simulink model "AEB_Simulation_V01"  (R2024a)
settings: Solver=ode23tb  StartTime=0.0  StopTime=inf  RelTol=2e-1
PreLoadFcn:
  | helperCreateDetectorBus;
model workspace (MAT data in the model file):
  EngPwr = 352122.842504
  EngWc = 4.047
  Tdiff = 849
  Tlim = 1000
  VEH : object (value not decoded)
undefined symbols (not defined in the file or in its folder): automotive_project_windows, blkdiag, C, car, D, Female, MATLAB, Performance, R2024a, Row, shared, sim3d_projects, Sim3dSensor, toolbox, UE, vector, VehicleSimulation, WindowsNoEditor
libraries: simulink x7, sim3dautolib x4, vehdynlibtirecommon x4, autolibutils x4, sharedtransform x2, sim3dcameralib x1, sim3dphyssensorlib x1, sim3dlib x1, motalgorithmslib x1, vehdynlibtire x1, vehdynlibsteering x1, autolibshared x1
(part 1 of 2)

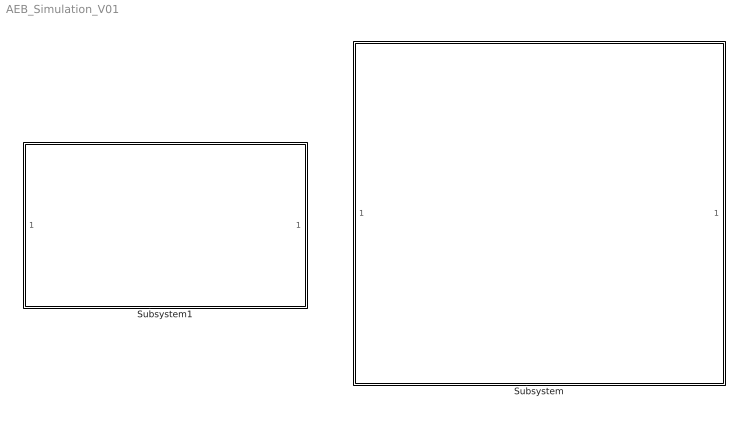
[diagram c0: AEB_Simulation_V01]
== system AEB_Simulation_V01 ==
  Subsystem : Subsystem
  Subsystem1 : Subsystem

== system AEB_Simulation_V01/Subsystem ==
  note: LED-Strip
  note: Controls
  {1..5} (5 alike) : LampBlock  LabelPosition=Hide
  Deceleration / Acceleration : SliderBlock  LabelPosition=Hide  ScaleMin=-1  ScaleMax=1  TickInterval=.25
  Direction : RotarySwitchBlock  LabelPosition=Hide
  Steering : KnobBlock  LabelPosition=Hide  ScaleMin=-400  ScaleMax=400  TickInterval=100
  Velocity : LinearGaugeBlock  LabelPosition=Hide  ScaleMax=30  TickInterval=5

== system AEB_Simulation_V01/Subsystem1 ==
  3D-Simulation : Subsystem
  AEB : Display
  BB-Detection and Tracking : Subsystem  Commented=on
  EGO : Subsystem
  MIO Detection : Subsystem  Commented=on
  Manual Switch : ManualSwitch  CurrentSetting=0
  Subsystem : Subsystem
  Terminator : Terminator
  Terminator1 : Terminator
  Terminator2 : Terminator
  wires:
  EGO/1(EGO_Position) -> 3D-Simulation/1(In1)
  Manual Switch/1 -> EGO/1(AEB), AEB/1
  MIO Detection/2(Relative Velocity) -> Terminator/1
  MIO Detection/4(MIO Track) -> Terminator2/1
  MIO Detection/3(Relative Distance) -> Terminator1/1
  MIO Detection/1(AEB) -> Manual Switch/1
  BB-Detection and Tracking/1(confirmedTracks) -> MIO Detection/1(confirmedTracks)
  3D-Simulation/1(lidar) -> Subsystem/1(In1), BB-Detection and Tracking/1(lidar)
  Subsystem/1(Out1) -> Manual Switch/2

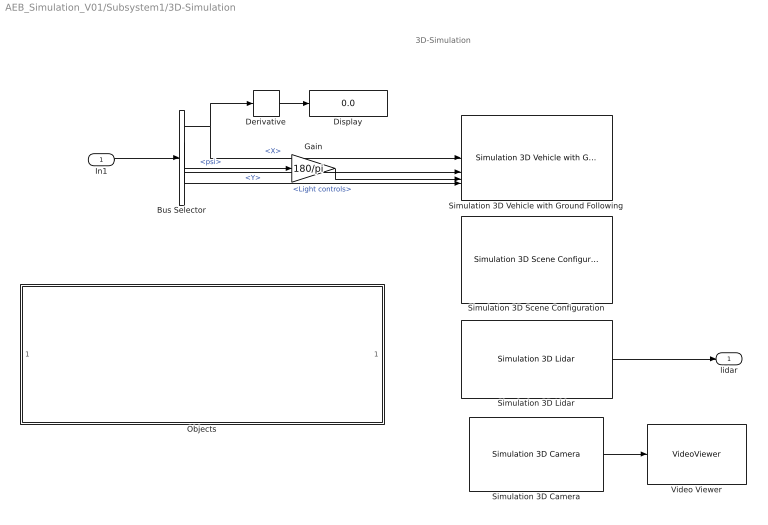
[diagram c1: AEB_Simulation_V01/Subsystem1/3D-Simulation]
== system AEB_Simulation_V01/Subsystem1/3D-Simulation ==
  note: 3D-Simulation
  In1 : Inport
  Bus Selector : BusSelector  OutputSignals=VehFdbk.InertFrm.Cg.Disp.X,VehFdbk.InertFrm.Cg.Disp.Y,VehFdbk.InertFrm.Cg.Ang.psi,Light controls
  Derivative : Derivative
  Display : Display
  Gain : Gain  Gain=180/pi
  Objects : Subsystem
  Simulation 3D Camera : sim3dcameralib/Simulation 3D Camera  Priority=1  sensorTag=Sim3dSensor�  sensorId=3  sensorName=Sim3dSensor�  vehTagList={'Scene Origin';'SimulinkVehicle1';'SimulinkVehicle2'}  vehTag=SimulinkVehicle1  mountLoc=Hood center  offsetFlag=on  tmountOffset=[-1.1, 0, 0.3]  extTmount=off  rmountOffset=[0, 5, 0]  extRmount=off  FocalLength=[1109, 1109]  OpticalCenter=[640, 360]  ImageSize=[720, 1280]  RadialDistortion=[0, 0]  TangentialDistortion=[0, 0]  SensorSkew=0  DepthOutportEnabled=off  SemanticOutportEnabled=off  TransformOutportEnabled=off  SampleTime=-1  mountPoint=[0.363999992609024 0 1.39999997615814]  mountOrientation=[0 -5 0]  aMode=3  ID=3
  Simulation 3D Lidar : sim3dphyssensorlib/Simulation 3D Lidar  Priority=1  sensorTag=Sim3dSensor�  sensorId=1  sensorName=Sim3dSensor�  vehTagList={'Scene Origin';'SimulinkVehicle1'}  vehTag=SimulinkVehicle1  mountLoc=Roof center  offsetFlag=off  tmountOffset=[0, 0, 0]  rmountOffset=[0, 0, 0]  DetectionRange=120  RangeResolution=0.02  VerticalFOV=40  VerticalResolution=1.25  HorizontalFOV=60  HorizontalResolution=0.16  DistanceOutportEnabled=off  ReflectivityOutportEnabled=off  SemanticOutportEnabled=off  TransformOutportEnabled=off  SampleTime=-1  mountPoint=[-0.449999988079071 0 1.67999994754791]  mountOrientation=[0 0 0]  aMode=3  ID=1
  Simulation 3D Scene Configuration : sim3dlib/Simulation 3D Scene Configuration  Priority=0  ProjectFormat=Default Scenes  SceneDesc=Parking lot  ProjectName=C:\MATLAB\R2024a\toolbox\shared\sim3d_projects\automotive_project_windows\UE\WindowsNoEditor\VehicleSimulation.exe  ScenePath=/Game/Maps/HwStrght  EnableOpenDRIVE=off  vehTagList={'Custom';'Scene Origin';'SimulinkVehicle1';'SimulinkVehicle2'}  vehTag=SimulinkVehicle1  FreeCameraInitialTranslation=[0, 0, 0]  FreeCameraDefaultInitialTranslation=[-6, 0, 2]  FreeCameraInitialRotation=[0, 0, 0]  FreeCameraDefaultInitialRotation=[0, -15, 0]  OpVisEn=off  Ts=0.1  EnableWindow=off  EnableRemoteAccess=off  EnableWeather=off  SunAzimuth=90  SunAltitude=40.0  EnableGeospatialSun=off  Latitude=0  Longitude=0  Date=2023-01-01  Time=10:30:00  GeoTimeZone=-5.0  SunDaylightSaving=off  wind=1  clouds=10  EnableVolumetricClouds=off  CloudCoverage=0  CloudAltitude=6  fog=0  rain=0  RaindropsEffect=off  SnowDensity=0  EnableGeospatial=off  UseTrueOrigin=off  OriginHeight=200  OriginLatitude=40.744652  OriginLongitude=-73.988864  MapStyle=Aerial  AdditionalAssetIDs=[]  UseAdvancedSunSky=off  SolarTime=11  TimeZone=-5  Day=21  Month=9  Year=2022  UseDaylightSavingTime=on  DSTStartDay=10  DSTStartMonth=3  DSTEndDay=3  DSTEndMonth=11  DSTSwitchHour=2  sensorTag=MainCamera1  sensorId=1  sensorName=MainCamera1  mountLoc=Origin  offsetFlag=off  tmountOffset=[0, 0, 0]  rmountOffset=[0, 0, 0]  HorizontalResolution=1280  VerticalResolution=720  HorizontalFOV=60  mountPoint=[0 0 0]  mountOrientation=[0 0 0]  aMode=3  ID=1  GeoTrigger=Inactive
  Simulation 3D Vehicle with Ground Following : sim3dautolib/Simulation 3D Vehicle with Ground Following  Priority=-1  PassVehMesh=Sedan  MeshPath=/MathWorksAutomotiveContent/Vehicles/Muscle/Meshes/SK_MuscleCar.SK_MuscleCar  TrackWidth=1.9  WheelBase=3  WheelRadius=0.35  VehColor=Red  InitialPos=[0, 0, 0]  InitialRot=[0, 0, 0]  ActorName=SimulinkVehicle1  SampleTime=-1  ActorType=SimulinkVehicle  ID=1  aMode=3  ActorTag=SimulinkVehicle1  CoordinateScheme=ISO  VehLightsControl=on  HeadlightColor=[ 1, 1, 1 ]  HighBeamIntensity=100000  LowBeamIntensity=60000  HighBeamConeAngle=70  LowBeamConeAngle=70  LeftHeadlightOrientation=[ 0, 0 ]  RightHeadlightOrientation=[ 0, 0 ]  BrakelightIntensity=500  ReverselightIntensity=500  SignallightIntensity=500  SignallightPeriod=1  SignalPulseWidth=50  TransformOutportEnabled=off
  Video Viewer : VideoViewer  FigPos=[593 850 943.333333333333 495.333333333333]
  lidar : Outport
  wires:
  Bus Selector/3 -> Gain/1  "<psi>"
  Bus Selector/2 -> Simulation 3D Vehicle with Ground Following/2  "<Y>"
  Bus Selector/4 -> Simulation 3D Vehicle with Ground Following/4  "<Light controls>"
  Simulation 3D Lidar/1 -> lidar/1
  Bus Selector/1 -> Derivative/1, Simulation 3D Vehicle with Ground Following/1  "<X>"
  In1/1 -> Bus Selector/1
  Gain/1 -> Simulation 3D Vehicle with Ground Following/3
  Derivative/1 -> Display/1
  Simulation 3D Camera/1 -> Video Viewer/1

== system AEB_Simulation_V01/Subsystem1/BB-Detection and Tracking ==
  note: Copyright 2019-2020 The MathWorks, Inc.
  note: Visualization
  note: Tracking Algorithm
  note: Lidar Segmentation and Clustering
  lidar : Inport
  Bounding Box Detector : MATLABSystem  System=HelperBoundingBoxDetectorBlock  DetectionBusName=detectionBus  SegmentationBusName=segmentationBus  NumLidarPoints=55000  XLimits=[ -70, 70 ]  YLimits=[ -6, 6 ]  ZLimits=[ -2, 10 ]  GroundMaxDistance=0.3  GroundReferenceVector=[ 0, 0, 1 ]  GroundMaxAngularDistance=5  SegmentationMinDistance=1.8  MinDetectionsPerCluster=1  MaxZDistanceCluster=3  MinZDistanceCluster=-3  EgoVehicleRadius=3  MeasurementNoise=blkdiag( 0.25*eye( 3 ), 25, eye( 3 ) )  MeasurementParameters="{  }"  SimulateUsing=Interpreted execution
  Calculate Detectability : MATLAB Function  TreatAsAtomicUnit=on
  Constant : Constant  Value=[1 3 6]
  Delay : Delay  DelayLength=1
  Terminator : Terminator
  Tracker : motalgorithmslib/Joint Probabilistic Data Association Multi Object Tracker  TrackerIndex=uint32( 0 )  FilterInitializationFcn=helperInitIMMFilter  MaxNumEvents=inf  EventGenerationFcn=jpdaEvents  MaxNumTracks=100  MaxNumSensors=20  TimeTolerance=1e-5  OOSMHandling=Terminate  MaxNumOOSMSteps=3  StateParametersSimulink=struct  HasStateParametersInput=off  EnableMemoryManagement=off  SimulateUsing=Interpreted execution  AssignmentThreshold=[75 1000]  InitializationThreshold=0  DetectionProbability=0.9  ClutterDensity=1e-9  TrackLogic=History  pHistoryConfThreshold=[7 10]  pHistoryDelThreshold=[8 10]  pIntegratedConfThreshold=0.95  pIntegratedDelThreshold=0.1  HitMissThreshold=0.1  NewTargetDensity=1e-5  DeathRate=0.01  TimeInputSource=Input port  HasCostMatrixInput=off  HasDetectableTrackIDsInput=on  TentativeTracksOutputPort=off  AllTracksOutputPort=on  InfoOutputPort=off  BusNameSource=Property  BusName=trackBus  BusName2Source=Auto  BusName2=BusTrackerInfo  MaxNumDetectionsPerSensor=100  MaxNumDetectionsPerCluster=5  MaxNumTracksPerCluster=5  ClusterViolationHandling=Split and warn
  Visualization : MATLABSystem  Commented=on  System=HelperLidarExampleDisplayBlock  LidarDataReaderBlockName=Lidar Data Reader  ImageDataReaderBlockName=Image Data Reader  DetectorBlockName=Bounding Box Detector  TrackerBlockName=Tracker  PositionIndex=[ 1, 3, 6 ]  VelocityIndex=[ 2, 4, 7 ]  DimensionIndex=[9 10 11]  YawIndex=8  RecordGIF=true  MovieName=myMovie  SimulateUsing=Interpreted execution
  confirmedTracks : Outport
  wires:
  Bounding Box Detector/1 -> Tracker/1
  Delay/1 -> Calculate Detectability/1(allTracks)
  Calculate Detectability/1(detectableTracksInput) -> Tracker/3
  Bounding Box Detector/2 -> Tracker/2
  Tracker/1 -> confirmedTracks/1
  Constant/1 -> Calculate Detectability/2(positionIndices)
  Tracker/2 -> Delay/1
  Bounding Box Detector/3 -> Terminator/1
  lidar/1 -> Bounding Box Detector/1

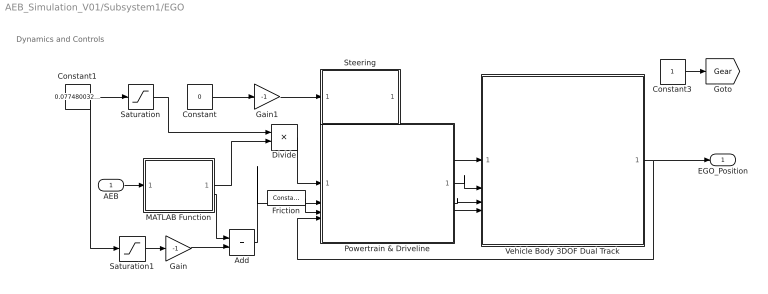
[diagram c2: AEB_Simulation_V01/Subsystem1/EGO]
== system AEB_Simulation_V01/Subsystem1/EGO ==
  note: Dynamics and Controls
  AEB : Inport
  Add : Sum
  Constant : Constant  Value=0
  Constant1 : Constant  Value=0.07748003246991852
  Constant3 : Constant
  Divide : Product  Inputs=**
  Friction : vehdynlibtirecommon/Constant  const=1  numWheels=4
  Gain : Gain  Gain=-1
  Gain1 : Gain  Gain=-1
  MATLAB Function : MATLAB Function  TreatAsAtomicUnit=on
  Powertrain & Driveline : Subsystem
  Saturation : Saturate  UpperLimit=1  LowerLimit=0
  Saturation1 : Saturate  UpperLimit=0  LowerLimit=-1
  Steering : Subsystem
  Vehicle Body 3DOF Dual Track : Subsystem
  EGO_Position : Outport
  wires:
  Gain/1 -> Add/2
  Constant3/1 -> [Gear]
  Powertrain & Driveline/2(Rear Force) -> Vehicle Body 3DOF Dual Track/3(FwR)
  Constant1/1 -> Saturation1/1, Saturation/1
  Constant/1 -> Gain1/1
  Powertrain & Driveline/3(DriverCmd) -> Vehicle Body 3DOF Dual Track/4(DriverCmd)
  Vehicle Body 3DOF Dual Track/1(VehFdbk) -> Powertrain & Driveline/4(VehFdbk), EGO_Position/1
  Powertrain & Driveline/1(Front Force) -> Vehicle Body 3DOF Dual Track/2(FwF)
  Steering/1(FrntWhl) -> Vehicle Body 3DOF Dual Track/1(WhlAngF)
  Friction/1 -> Powertrain & Driveline/3(Friction)
  Saturation1/1 -> Gain/1
  Saturation/1 -> Divide/1
  Gain1/1 -> Steering/1(HndWhl)
  Add/1 -> Powertrain & Driveline/2(Decel)
  MATLAB Function/1(acc) -> Divide/2
  MATLAB Function/2(dec) -> Add/1
  Divide/1 -> Powertrain & Driveline/1(Acc)
  AEB/1 -> MATLAB Function/1(AEB)

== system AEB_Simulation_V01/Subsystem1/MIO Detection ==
  confirmedTracks : Inport
  AEB Calculation : Subsystem
  Constant : Constant  Value=0
  Find Obstacle : MATLAB Function  TreatAsAtomicUnit=on
  Most Important Object (MIO) : Display
  Position Selector : Constant  Value=[1 0 0 0 0 0;0 0 1 0 0 0]
  AEB : Outport  VectorParamsAs1DForOutWhenUnconnected=off
  Relative Velocity : Outport  Port=2  VectorParamsAs1DForOutWhenUnconnected=off
  Relative Distance : Outport  Port=3  VectorParamsAs1DForOutWhenUnconnected=off
  MIO Track : Outport  Port=4  VectorParamsAs1DForOutWhenUnconnected=off
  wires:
  Position Selector/1 -> Find Obstacle/3(positionSelector)
  Find Obstacle/2(vx) -> Relative Velocity/1
  Find Obstacle/3(mioTrack) -> AEB Calculation/1(In1), Most Important Object (MIO)/1, MIO Track/1
  Constant/1 -> Find Obstacle/2(curvature)
  confirmedTracks/1 -> Find Obstacle/1(confirmedTracks)
  Find Obstacle/1(x) -> Relative Distance/1  "relative_distance"
  AEB Calculation/1(AEB) -> AEB/1

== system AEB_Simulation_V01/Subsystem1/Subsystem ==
  In1 : Inport
  AEB_01 : Subsystem
  Data Type Conversion : DataTypeConversion
  Data Type Conversion1 : DataTypeConversion
  Out1 : Outport
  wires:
  AEB_01/1(AEB) -> Data Type Conversion1/1
  Data Type Conversion/1 -> AEB_01/1(lidar)
  In1/1 -> Data Type Conversion/1
  Data Type Conversion1/1 -> Out1/1

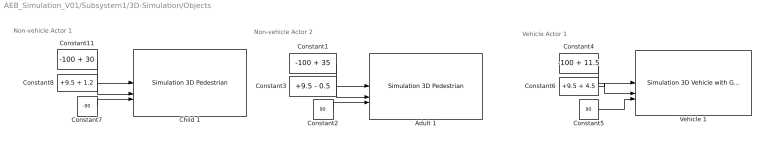
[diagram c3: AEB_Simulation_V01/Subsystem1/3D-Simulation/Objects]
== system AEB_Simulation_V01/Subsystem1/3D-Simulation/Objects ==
  note: Non-vehicle Actor 1
  note: Non-vehicle Actor 2
  note: Vehicle Actor 1
  Adult 1 : sim3dautolib/Simulation 3D Pedestrian  Priority=-1  PedestrianType=Female 3  Scale=[1, 1, 1]  InitialPos=[10, 0, 0]  InitialYaw=0  ActorName=SimulinkPedestrian2  SampleTime=-1  ActorType=SimulinkPedestrian  ActorTag=SimulinkPedestrian2  ID=2  aMode=3  CoordinateScheme=ISO  TransformOutportEnabled=off
  Child 1 : sim3dautolib/Simulation 3D Pedestrian  Priority=-1  PedestrianType=Child  Scale=[1, 1, 1]  InitialPos=[0, 0, 0]  InitialYaw=0  ActorName=SimulinkPedestrian1  SampleTime=-1  ActorType=SimulinkPedestrian  ActorTag=SimulinkPedestrian1  ID=1  aMode=3  CoordinateScheme=ISO  TransformOutportEnabled=off
  Constant1 : Constant  Value=-100 + 35
  Constant11 : Constant  Value=-100 + 30
  Constant2 : Constant  Value=90
  Constant3 : Constant  Value=+9.5 - 0.5
  Constant4 : Constant  Value=-100 + 11.5
  Constant5 : Constant  Value=90
  Constant6 : Constant  Value=+9.5 + 4.5
  Constant7 : Constant  Value=-90
  Constant8 : Constant  Value=+9.5 + 1.2
  Vehicle 1 : sim3dautolib/Simulation 3D Vehicle with Ground Following  Priority=-1  PassVehMesh=Sedan  MeshPath=/MathWorksAutomotiveContent/Vehicles/Muscle/Meshes/SK_MuscleCar.SK_MuscleCar  TrackWidth=1.9  WheelBase=3  WheelRadius=0.35  VehColor=Orange  InitialPos=[0, 0, 0]  InitialRot=[0, 0, 90]  ActorName=SimulinkVehicle2  SampleTime=-1  ActorType=SimulinkVehicle  ID=2  aMode=3  ActorTag=SimulinkVehicle2  CoordinateScheme=ISO  VehLightsControl=off  HeadlightColor=[ 1, 1, 1 ]  HighBeamIntensity=100000  LowBeamIntensity=60000  HighBeamConeAngle=70  LowBeamConeAngle=70  LeftHeadlightOrientation=[ 0, 0 ]  RightHeadlightOrientation=[ 0, 0 ]  BrakelightIntensity=500  ReverselightIntensity=500  SignallightIntensity=500  SignallightPeriod=1  SignalPulseWidth=50  TransformOutportEnabled=off
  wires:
  Constant8/1 -> Child 1/2
  Constant7/1 -> Child 1/3
  Constant11/1 -> Child 1/1
  Constant3/1 -> Adult 1/2
  Constant1/1 -> Adult 1/1
  Constant2/1 -> Adult 1/3
  Constant4/1 -> Vehicle 1/1
  Constant6/1 -> Vehicle 1/2
  Constant5/1 -> Vehicle 1/3

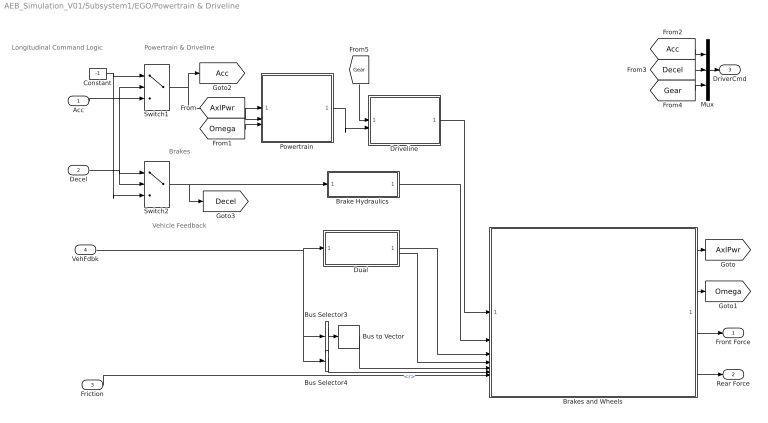
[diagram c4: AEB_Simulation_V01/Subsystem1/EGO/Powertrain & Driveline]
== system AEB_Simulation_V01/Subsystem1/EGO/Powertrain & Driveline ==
  note: Longitudinal Command Logic
  note: Brakes
  note: Powertrain & Driveline
  note: Vehicle Feedback
  Acc : Inport
  Decel : Inport  Port=2
  Friction : Inport  Port=3
  VehFdbk : Inport  Port=4
  Brake Hydraulics : Subsystem
  Brakes and Wheels : Subsystem  TreatAsAtomicUnit=on
  Bus Selector3 : BusSelector  OutputSignals=VehFdbk.BdyFrm.FrntAxl.Steer.WhlAngFL,VehFdbk.BdyFrm.FrntAxl.Steer.WhlAngFR,VehFdbk.BdyFrm.RearAxl.Steer.WhlAngRL,VehFdbk.BdyFrm.RearAxl.Steer.WhlAngRR  OutputAsBus=on
  Bus Selector4 : BusSelector  OutputSignals=VehFdbk.BdyFrm.Cg.AngVel.r
  Bus to Vector : BusToVector
  Constant : Constant  Value=-1
  Driveline : Subsystem  Variant=on  VariantControlMode=label  VariantControl=Variant1  LabelModeActiveChoice=1
  Dual : Subsystem  VariantControl=1
  Mux : Mux  Inputs=3
  Powertrain : Subsystem
  Switch1 : Switch  Criteria=u2 > Threshold
  Switch2 : Switch  Criteria=u2 > Threshold
  Front Force : Outport  VectorParamsAs1DForOutWhenUnconnected=off
  Rear Force : Outport  Port=2  VectorParamsAs1DForOutWhenUnconnected=off
  DriverCmd : Outport  Port=3  VectorParamsAs1DForOutWhenUnconnected=off
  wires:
  Decel/1 -> Switch1/2, Switch2/2, Switch2/1
  Acc/1 -> Switch1/3
  Constant/1 -> Switch2/3, Switch1/1
  Bus Selector3/1 -> Bus to Vector/1
  Switch1/1 -> [Acc], Powertrain/1(Acc)
  Powertrain/1(AxlTrq) -> Driveline/2(TPowertrain)
  [AxlPwr] -> Powertrain/2(AxlPwr)
  [Omega] -> Powertrain/3(Omega)
  Switch2/1 -> [Decel], Brake Hydraulics/1(BrkPrsCmd)
  Friction/1 -> Brakes and Wheels/7(Friction)
  VehFdbk/1 -> Bus Selector4/1, Bus Selector3/1, Dual/1(VehFdbk)
  Brakes and Wheels/2(Omega) -> [Omega]
  Brakes and Wheels/3(FrontF) -> Front Force/1
  Brakes and Wheels/4(RearF) -> Rear Force/1
  Brakes and Wheels/1(AxlPwr) -> [AxlPwr]
  Bus to Vector/1 -> Brakes and Wheels/5(WhlAng)
  Dual/2(Fz) -> Brakes and Wheels/4(Fz)
  Bus Selector4/1 -> Brakes and Wheels/6(YawRate)  "<r>"
  Brake Hydraulics/1(BrkPrs) -> Brakes and Wheels/2(BrkPrs)
  Driveline/1(TAxles) -> Brakes and Wheels/1(AxlTrq)
  Dual/1(VehVel) -> Brakes and Wheels/3(VehVel)
  Mux/1 -> DriverCmd/1
  [Acc] -> Mux/1
  [Decel] -> Mux/2
  [Gear] -> Mux/3
  [Gear] -> Driveline/1(Gear)

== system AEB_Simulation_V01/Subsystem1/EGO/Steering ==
  HndWhl : Inport
  Kinematic Steering : vehdynlibsteering/Kinematic Steering  StrgType=Rack and pinion  StrgRatioType=Constant  Loc=Front  NrmlFctr=0.01  TrckWdth=1.4  WhlBase=1.524  Db=0  StrgRng=(pi/180)*470  StrgAngBpts="[-6.2832   -5.0265   -3.7699   -2.5133   -1.2566         0    1.2566    2.5133    3.7699    5.0265    6.2832]"  StrgRatioTbl="[13.5000   13.3750   13.2500   13.1250   13.0000   13.0000   13.0000   13.1250   13.2500   13.3750   13.5000 ]"  StrgRatio=100  PctAckIn=off  PctAck=100  PctAckTbl=ones(1,11)*100  StrgArmLngth=0.1  RckCsLngth=0.5  TieRodLngth=.4  D=0.2  PnnRadius=0.0057  PnnRadiusTbl="[0.0055    0.0055    0.0056    0.0057    0.0058    0.0057    0.0057    0.0057    0.0056    0.0055    0.0055]"  RodLngth=0.1  ParaArmLngth=0.9  aMode=2
  Mux : Mux  Inputs=2
  Signal Specification : SignalSpecification  Unit=deg
  Terminator6 : Terminator
  Unit Conversion : UnitConversion
  FrntWhl : Outport  VectorParamsAs1DForOutWhenUnconnected=off
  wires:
  Signal Specification/1 -> Unit Conversion/1
  Kinematic Steering/1 -> Terminator6/1
  HndWhl/1 -> Signal Specification/1
  Kinematic Steering/2 -> Mux/1
  Kinematic Steering/3 -> Mux/2
  Unit Conversion/1 -> Kinematic Steering/1
  Mux/1 -> FrntWhl/1

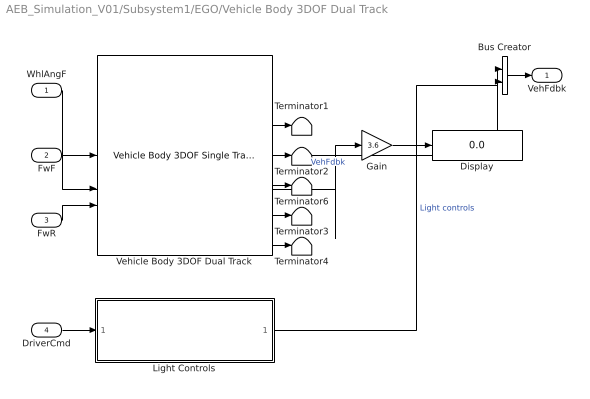
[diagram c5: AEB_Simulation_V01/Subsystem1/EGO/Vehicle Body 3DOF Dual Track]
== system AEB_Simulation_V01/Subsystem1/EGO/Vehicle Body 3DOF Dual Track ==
  WhlAngF : Inport
  FwF : Inport  Port=2
  FwR : Inport  Port=3
  DriverCmd : Inport  Port=4
  Bus Creator : BusCreator  Inputs=2
  Display : Display
  Gain : Gain  Gain=3.6
  Light Controls : Subsystem
  Terminator{1..4,6} (5 alike) : Terminator
  Vehicle Body 3DOF Dual Track : autolibshared/Vehicle Body 3DOF Single Track  trackMode=Dual  inputMode=External forces  frontSteerMode=on  rearSteerMode=off  windMode=off  muMode=off  extFMode=off  extMMode=off  htchFMode=off  htchMMode=off  extXo=off  extpsio=off  extxdoto=off  extro=off  extYo=off  extTamb=off  extydoto=off  aMode=2  NF=2  NR=2  m=1500  a=1.4  b=1.6  h=0.35  dh=1  hh=0.2  X_o=-100  xdot_o=0  CalphaMode=off  sigmaMode=on  d=0  hl=0  w=[1.4,1.4]  Cy_f=12e3  Cy_r=11e3  sigma_f=.1  sigma_r=.1  alpha_f_brk=[-.1 .1]  Cy_f_data=[-9e3 9e3]  alpha_r_brk=[-.1 .1]  Cy_r_data=[-9e3 9e3]  Y_o=+9.5  ydot_o=0  Izz=2000  psi_o=0  r_o=0  Af=2  Cd=.3  Cl=.1  Cpm=.1  beta_w=[0:0.01:0.3]  Cs=[0:0.03:0.9]  Cym=[0:0.01:0.3]  Pabs=101325  Tair=273  g=9.81  mu=1  xdot_tol=.1  Fznom=5000  Fxtire_sat=7e4  Fytire_sat=7e4  longOff=0  latOff=0  vertOff=0  wrapAng=off
  VehFdbk : Outport
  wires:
  Vehicle Body 3DOF Dual Track/6 -> Terminator3/1
  Vehicle Body 3DOF Dual Track/3 -> Terminator1/1
  Vehicle Body 3DOF Dual Track/4 -> Terminator2/1
  Vehicle Body 3DOF Dual Track/7 -> Terminator4/1
  Vehicle Body 3DOF Dual Track/1 -> Bus Creator/1  "VehFdbk"
  FwF/1 -> Vehicle Body 3DOF Dual Track/2
  WhlAngF/1 -> Vehicle Body 3DOF Dual Track/1
  FwR/1 -> Vehicle Body 3DOF Dual Track/3
  DriverCmd/1 -> Light Controls/1(DriverCmd)
  Light Controls/1(Light Controls) -> Bus Creator/2  "Light controls"
  Bus Creator/1 -> VehFdbk/1
  Vehicle Body 3DOF Dual Track/2 -> Gain/1
  Vehicle Body 3DOF Dual Track/5 -> Terminator6/1
  Gain/1 -> Display/1

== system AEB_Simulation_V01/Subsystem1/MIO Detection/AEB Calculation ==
  In1 : Inport
  Demux : Demux  Outputs=11
  MATLAB Function : MATLAB Function  TreatAsAtomicUnit=on
  th_AEB : Constant  Value=[20, 15, 10]
  AEB : Outport  VectorParamsAs1DForOutWhenUnconnected=off
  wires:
  Demux/3 -> ?
  MATLAB Function/1(AEB) -> AEB/1
  Demux/1 -> MATLAB Function/1(x_obj)
  In1/1 -> Demux/1
  Demux/5 -> ?
  Demux/6 -> ?
  Demux/2 -> ?
  Demux/4 -> ?
  Demux/7 -> ?
  Demux/11 -> ?
  Demux/8 -> ?
  Demux/9 -> ?
  Demux/10 -> ?
  th_AEB/1 -> MATLAB Function/2(th_AEB)

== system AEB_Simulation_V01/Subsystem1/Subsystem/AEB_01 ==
  lidar : Inport
  Constant2 : Constant  Value=0
  Data Type Conversion1 : DataTypeConversion
  Display1 : Display
  Display2 : Display
  Display3 : Display
  MATLAB System : MATLABSystem  System=AEBLid_ObjectDetection_Var_C_V01  steeringFactor=470 / 36  lanewidth=2.1  wheelbase=2.565  hoodOffset=2.565 / 3  simulationtime=2.5  dt=0.25  BoundingBox=[ 0.1, 0.8, 0.1, 0.8, 0.6, 2.5 ]  p1_x=[0.0 1.5 1.5 0.0 -1.5 -1.5 0]  p1_y=[0.0 0.0 8.0 10.0 8.0 0.0 0.0]
  AEB : Outport
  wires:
  Data Type Conversion1/1 -> Display3/1
  Constant2/1 -> MATLAB System/2
  lidar/1 -> MATLAB System/1
  MATLAB System/3 -> Display2/1
  MATLAB System/2 -> Data Type Conversion1/1
  MATLAB System/1 -> AEB/1, Display1/1

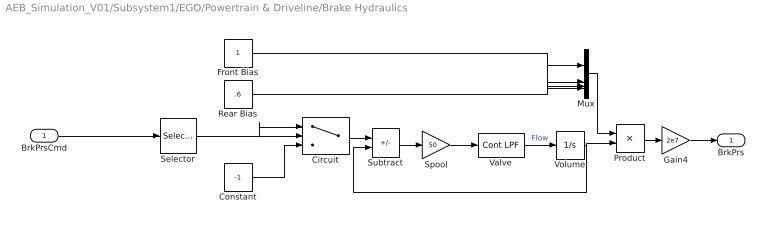
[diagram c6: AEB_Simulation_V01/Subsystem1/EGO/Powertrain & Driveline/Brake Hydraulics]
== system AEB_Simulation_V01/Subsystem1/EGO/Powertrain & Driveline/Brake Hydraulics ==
  BrkPrsCmd : Inport
  Circuit : Switch  Criteria=u2 ~= 0
  Constant : Constant  Value=-1
  Front Bias : Constant
  Gain4 : Gain  Gain=2e7
  Mux : Mux
  Product : Product
  Rear Bias : Constant  Value=.6
  Selector : Selector  InputPortWidth=1  IndexOptions=Index vector (dialog)  Indices=[1 1 1 1]  OutputSizes=1
  Spool : Gain  Gain=50
  Subtract : Sum  Inputs=+-
  Valve : autolibutils/Cont LPF  wc=20*2*pi  AbsoluteTolerance=auto  aMode=2
  Volume : Integrator  LimitOutput=on  UpperSaturationLimit=1  LowerSaturationLimit=0
  BrkPrs : Outport  VectorParamsAs1DForOutWhenUnconnected=off
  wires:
  Volume/1 -> Subtract/2, Product/2
  Valve/1 -> Volume/1  "Flow"
  BrkPrsCmd/1 -> Selector/1
  Gain4/1 -> BrkPrs/1
  Circuit/1 -> Subtract/1
  Constant/1 -> Circuit/3
  Subtract/1 -> Spool/1
  Spool/1 -> Valve/1
  Front Bias/1 -> Mux/2, Mux/1
  Rear Bias/1 -> Mux/3, Mux/4
  Product/1 -> Gain4/1
  Mux/1 -> Product/1
  Selector/1 -> Circuit/1, Circuit/2

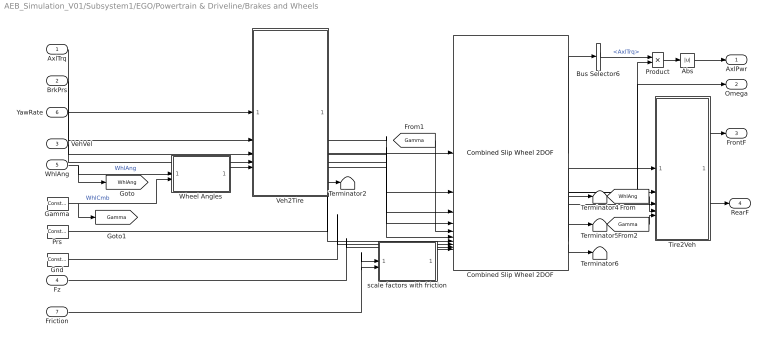
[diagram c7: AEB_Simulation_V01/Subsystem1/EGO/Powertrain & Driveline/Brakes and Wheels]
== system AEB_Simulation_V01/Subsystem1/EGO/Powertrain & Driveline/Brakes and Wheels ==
  AxlTrq : Inport
  BrkPrs : Inport  Port=2
  VehVel : Inport  Port=3
  Fz : Inport  Port=4  PortDimensions=4
  WhlAng : Inport  Port=5
  YawRate : Inport  Port=6
  Friction : Inport  Port=7
  Abs : Abs
  Bus Selector6 : BusSelector  OutputSignals=AxlTrq
  Combined Slip Wheel 2DOF : vehdynlibtire/Combined Slip Wheel 2DOF  tireType=Performance car 225/40R19  BrakeType=Disc  vertType=Magic Formula  plySteer=off  turnslip=off  mu_static=.3  mu_kinetic=.2  disk_abore=.05  Rm=.177  num_pads=2  drum_abore=0.0508  drum_a=0.123  drum_c=0.212  drum_r=0.15  drum_theta1=0  drum_theta2=126  brake_p_bpt=[1 11.4736842105263 21.9473684210526 32.4210526315789 42.8947368421053 53.3684210526316 63.8421052631579 74.3157894736842 84.7894736842105 95.2631578947368 105.736842105263 116.210526315789 126.684210526316 137.157894736842 147.631578947368 158.105263157895 168.578947368421 179.052631578947 189.526315789474 200]  brake_n_bpt=[0 52.6315789473684 105.263157894737 157.894736842105 210.526315789474 263.157894736842 315.789473684211 368.421052631579 421.052631578947 473.684210526316 526.315789473684 578.947368421053 631.578947368421 684.210526315789 736.842105263158 789.473684210526 842.105263157895 894.736842105263 947.368421052632 1000]  f_brake_t=[43.4900602404453 42.5056030554862 41.5350898940194 40.5780454442085 39.6340111501808 38.7025443887544 37.7832176914519 36.8756180088306 35.9793460143796 35.0940154454303 34.2192524787115 33.3546951383474 32.4999927342521 31.6548053290159 30.8188032315107 29.991666515561 29.1730845621415 28.362755623661 27.5603864089927 26.765691687993;498.991217495636 487.695866636631 476.560505099801 465.5796793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  tireParamSet=vdynPassCar.mat  PRESMAX=1000000  PRESMIN=10000  FZMAX=9200  FZMIN=100  VXLOW=.01  KPUMAX=1.5  KPUMIN=-1.5  ALPMAX=1.5  ALPMIN=-1.5  CAMMAX=0.17453  CAMMIN=-0.17453  LONGVL=16.7  FxRelFreqLwrLim=200*pi  FyRelFreqLwrLim=200*pi  MyRelFreqLwrLim=100*pi  omegao=0  br=1e-3  UNLOADED_RADIUS=0.33136  NOMPRES=262000  FNOMIN=4600  WIDTH=0.225  RIM_RADIUS=0.2413  MASS=10.35  IYY=0.99  GRAVITY=-9.81  zo=0  zdoto=0  BREFF=8.25094594147963  DREFF=0.260468730454265  FREFF=0.0735298544471851  Q_RE0=1.00866439868088  Q_V1=0.000760413786224011  Q_V2=0.0463384792019201  Q_FZ1=0  Q_FZ2=15.6870832810226  Q_FZ3=0  Q_FCX=0.138643970247602  Q_FCY=0.10843499565426  Q_FCY2=-0.465763352339538  PFZ1=0.69958166705601  VERTICAL_STIFFNESS=207885.061134007  VERTICAL_DAMPING=494.649255786991  BOTTOM_OFFST=.01  BOTTOM_STIFF=2e6  LONGITUDINAL_STIFFNESS=388714.175879854  LATERAL_STIFFNESS=157087.404633332  PCFX1=0.18539229191199  PCFX2=0  PCFX3=0  PCFY1=0.163183345037677  PCFY2=0  PCFY3=0.249094918231954  Q_RA1=0.675942571700787  Q_RA2=0.73800463546164  Q_RB1=1.04487486456705  Q_RB2=-1.191763806629  PCX1=1.58523057950359  PDX1=1.0239116238178  PDX2=-0.0842405110022724  PDX3=0  PEX1=0.110312777158455  PEX2=0.313468516038146  PEX3=0  PEX4=0.0016060905760045  PKX1=21.3872544684023  PKX2=14.0006541873175  PKX3=-0.405326109653452  PHX1=0.000212599305364818  PHX2=0.00115950515263055  PVX1=1.59236164471432e-05  PVX2=0.000104321112127671  PPX1=-0.349461321276586  PPX2=0.387840040616429  PPX3=-0.0969947336569324  PPX4=0.0632271859795801  RBX1=12.7633329850276  RBX2=9.5787123658471  RBX3=0  RCX1=1.02796280922059  REX1=-0.45202516851367  REX2=-0.47304886171176  RHX1=0.000233272373115809  QSX1=-0.00788307788961443  QSX2=0.954629515459396  QSX3=0.0155855777667025  QSX4=0.125904607142414  QSX5=1.01110069703963  QSX6=20.1938577118433  QSX7=0.310818120717083  QSX8=-0.0430823751139655  QSX9=0.636494404888216  QSX10=0.142438060591663  QSX11=0.346766530036373  QSX12=0  QSX13=0  QSX14=0  PPMX1=0  PCY1=1.34299950037631  PDY1=0.878267729082195  PDY2=-0.0644597923147385  PDY3=0  PEY1=-0.809776534470972  PEY2=-0.600180598867198  PEY3=0.0991732552633487  PEY4=-6.5577974035573  PEY5=0  PKY1=-15.5714726518315  PKY2=1.73126522291751  PKY3=0.365349873517229  PKY4=1.98176755955416  PKY5=0  PKY6=-0.884005199550313  PKY7=-0.237259727611847  PHY1=-0.00183370557235628  PHY2=0.00346401302716671  PVY1=-0.00675427560163264  PVY2=0.036379218103843  PVY3=-0.163543984089166  PVY4=-0.491003349625726  PPY1=-0.62059646553185  PPY2=-0.0647824842338686  PPY3=-0.164648843290686  PPY4=0.283193909060098  PPY5=0  RBY1=10.7588809173639  RBY2=7.70420065295029  RBY3=3.40283755070691e-06  RBY4=0  RCY1=1.06691874059059  REY1=0.308244924574305  REY2=7.48775032604508e-06  RHY1=0.0118479204960415  RHY2=7.63650177161071e-06  RVY1=0.0560024425050078  RVY2=7.48487127056197e-06  RVY3=0  RVY4=98.4047026517149  RVY5=2.02759273900054  RVY6=15.7623064923347  QSY1=0.00699077564863536  QSY2=0  QSY3=0.00153535478298811  QSY4=8.55710322455322e-05  QSY5=0  QSY6=0  QSY7=0.89443879773793  QSY8=-0.403227641260894  QBZ1=11.666656027484  QBZ2=-1.30355438574485  QBZ3=0  QBZ4=0.177918305399071  QBZ5=-0.162481135068033  QBZ6=0  QBZ9=30.1445534682089  QBZ10=0  QCZ1=1.29026978207574  QDZ1=0.0886972644991399  QDZ2=-0.0058634820161856  QDZ3=0.3805597481383  QDZ4=0  QDZ6=0.00160914918118959  QDZ7=-0.00211036330862154  QDZ8=-0.13921904912557  QDZ9=0.00816585550028243  QDZ10=0  QDZ11=0  QEZ1=-2.19802254534746  QEZ2=1.01850535789165  QEZ3=0  QEZ4=0.278379679112054  QEZ5=-0.548414722765386  QHZ1=0.00148361198869669  QHZ2=0.00202017567585904  QHZ3=0.240316641332066  QHZ4=-0.210114035738085  PPZ1=-0.443927982388615  PPZ2=0  SSZ1=0.00914999585397887  SSZ2=0.0389830656052735  SSZ3=0  SSZ4=0  PDXP1=0.396718274678791  PDXP2=0  PDXP3=0  PKYP1=1.00587060633573  PDYP1=0.40483048923438  PDYP2=0  PDYP3=0  PDYP4=0  PHYP1=0.992731942067188  PHYP2=0.150352945499914  PHYP3=0  PHYP4=-3.98988682633674  PECP1=0.502379254513503  PECP2=0  QDTP1=10.0178654287947  QCRP1=0.200627747200702  QCRP2=0.0995735881599772  QBRP1=0.0997107127960717  QDRP1=1.01432910167423  QDRP2=0  aMode=2
  Gamma : vehdynlibtirecommon/Constant  const=0  numWheels=4
  Gnd : vehdynlibtirecommon/Constant  const=0  numWheels=4
  Product : Product
  Prs : vehdynlibtirecommon/Constant  const=2.4e5  numWheels=4
  Terminator{2,4..6} (4 alike) : Terminator
  Tire2Veh : Subsystem
  Veh2Tire : Subsystem
  Wheel Angles : Subsystem
  scale factors with friction : Subsystem  mask{numWheels=4}
      mask prompts: numWheels "Number of wheels"
  AxlPwr : Outport
  Omega : Outport  Port=2
  FrontF : Outport  Port=3
  RearF : Outport  Port=4
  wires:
  Gnd/1 -> Combined Slip Wheel 2DOF/8
  Combined Slip Wheel 2DOF/1 -> Bus Selector6/1
  Combined Slip Wheel 2DOF/2 -> Omega/1, Product/2
  Combined Slip Wheel 2DOF/7 -> Terminator5/1
  Combined Slip Wheel 2DOF/6 -> Terminator4/1
  Product/1 -> Abs/1
  Fz/1 -> Combined Slip Wheel 2DOF/9
  Veh2Tire/3(xdotAxle) -> Combined Slip Wheel 2DOF/3
  Combined Slip Wheel 2DOF/8 -> Terminator6/1
  Prs/1 -> Combined Slip Wheel 2DOF/7
  Friction/1 -> scale factors with friction/1(lamda_mu_x), scale factors with friction/2(lamda_mu_y)
  Abs/1 -> AxlPwr/1
  Bus Selector6/1 -> Product/1  "<AxlTrq>"
  scale factors with friction/1(lambdas) -> Combined Slip Wheel 2DOF/10
  Veh2Tire/5(psidot) -> Combined Slip Wheel 2DOF/6
  Combined Slip Wheel 2DOF/3 -> Tire2Veh/1(Fx)
  Combined Slip Wheel 2DOF/4 -> Tire2Veh/2(Fy)
  Combined Slip Wheel 2DOF/5 -> Tire2Veh/3(Fz)
  WhlAng/1 -> [WhlAng], Wheel Angles/1(steer)  "WhlAng"
  Gamma/1 -> [Gamma], Wheel Angles/2(camber)  "WhlCmb"
  Tire2Veh/1(FxyF) -> FrontF/1
  Tire2Veh/2(FxyR) -> RearF/1
  Veh2Tire/2(T) -> Combined Slip Wheel 2DOF/2
  BrkPrs/1 -> Veh2Tire/2(BrkPrs)
  AxlTrq/1 -> Veh2Tire/1(AxlTrq)
  Wheel Angles/1(WhlAngB) -> Veh2Tire/5(WhlAng)
  VehVel/1 -> Veh2Tire/4(VehVel)
  Veh2Tire/6(zdotAxle) -> Terminator2/1
  Veh2Tire/1(P) -> Combined Slip Wheel 2DOF/1
  Veh2Tire/4(ydotAxle) -> Combined Slip Wheel 2DOF/4
  YawRate/1 -> Veh2Tire/3(r)
  [WhlAng] -> Tire2Veh/4(WhlAng)
  [Gamma] -> Combined Slip Wheel 2DOF/5
  [Gamma] -> Tire2Veh/5(WhlCmb)

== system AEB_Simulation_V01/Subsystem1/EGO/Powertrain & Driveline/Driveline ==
  Gear : Inport
  TPowertrain : Inport  Port=2  PortDimensions=1
  AWD : Subsystem  VariantControl=2
  FWD : Subsystem  VariantControl=1
  RWD : Subsystem  VariantControl=0
  TAxles : Outport  PortDimensions=4  VectorParamsAs1DForOutWhenUnconnected=off

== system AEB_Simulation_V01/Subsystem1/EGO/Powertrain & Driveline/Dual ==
  VehFdbk : Inport
  Dual Fz : Subsystem
  Dual V : Subsystem
  VehVel : Outport  VectorParamsAs1DForOutWhenUnconnected=off
  Fz : Outport  Port=2  VectorParamsAs1DForOutWhenUnconnected=off
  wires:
  Dual V/1(Out1) -> VehVel/1
  VehFdbk/1 -> Dual Fz/1(In1), Dual V/1(In1)
  Dual Fz/1(Out1) -> Fz/1

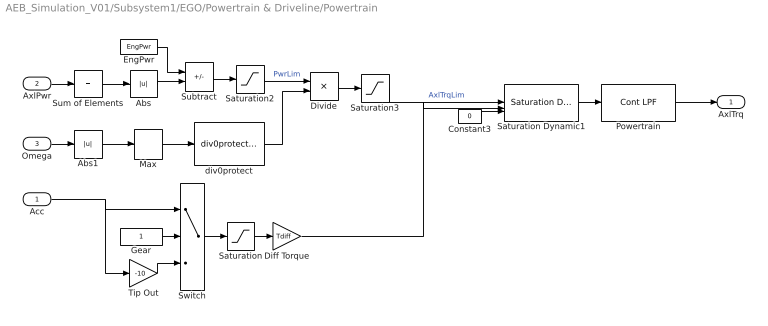
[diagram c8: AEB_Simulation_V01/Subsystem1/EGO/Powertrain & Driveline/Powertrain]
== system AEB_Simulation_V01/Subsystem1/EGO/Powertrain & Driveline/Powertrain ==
  Acc : Inport
  AxlPwr : Inport  Port=2  PortDimensions=4
  Omega : Inport  Port=3  PortDimensions=4
  Abs : Abs  ZeroCross=off
  Abs1 : Abs  ZeroCross=off
  Constant3 : Constant  Value=0
  Diff Torque : Gain  Gain=Tdiff
  Divide : Product  Inputs=*/
  EngPwr : Constant  Value=EngPwr
  Gear : Constant  SampleTime=-1
  Max : MinMax  Function=max  ZeroCross=off
  Powertrain : autolibutils/Cont LPF  wc=EngWc  AbsoluteTolerance=auto  aMode=2
  Saturation : Saturate  UpperLimit=inf  LowerLimit=0  ZeroCross=off
  Saturation Dynamic1 : simulink/Discontinuities/Saturation Dynamic  OutMin=[]  OutMax=[]  OutDataTypeStr=Inherit: Same as second input  OutDataType=fixdt(1, 16)  OutScaling=2^-10  DoSatur=off
  Saturation2 : Saturate  UpperLimit=inf  LowerLimit=100  ZeroCross=off
  Saturation3 : Saturate  UpperLimit=Tlim  LowerLimit=0  ZeroCross=off
  Subtract : Sum  Inputs=+-
  Sum of Elements : Sum  Inputs=+
  Switch : Switch  ZeroCross=off
  Tip Out : Gain  Gain=-10
  div0protect : autolibutils/div0protect - poly  thresh=1  ZeroCross1=on  aMode=2
  AxlTrq : Outport  VectorParamsAs1DForOutWhenUnconnected=off
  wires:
  Powertrain/1 -> AxlTrq/1
  Switch/1 -> Saturation/1
  Acc/1 -> Tip Out/1, Switch/1
  Saturation/1 -> Diff Torque/1
  Diff Torque/1 -> Saturation Dynamic1/2
  Gear/1 -> Switch/2
  Saturation Dynamic1/1 -> Powertrain/1
  Tip Out/1 -> Switch/3
  Constant3/1 -> Saturation Dynamic1/3
  Sum of Elements/1 -> Abs/1
  Abs/1 -> Subtract/2
  Divide/1 -> Saturation3/1
  div0protect/1 -> Divide/2
  Omega/1 -> Abs1/1
  Subtract/1 -> Saturation2/1
  Saturation2/1 -> Divide/1  "PwrLim"
  EngPwr/1 -> Subtract/1
  AxlPwr/1 -> Sum of Elements/1
  Saturation3/1 -> Saturation Dynamic1/1  "AxlTrqLim"
  Max/1 -> div0protect/1
  Abs1/1 -> Max/1

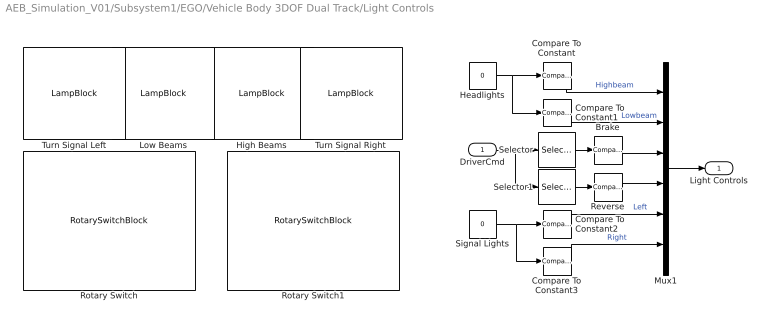
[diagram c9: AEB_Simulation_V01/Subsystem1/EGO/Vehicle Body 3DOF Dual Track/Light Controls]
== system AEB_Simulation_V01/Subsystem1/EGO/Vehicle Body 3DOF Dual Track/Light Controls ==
  DriverCmd : Inport
  Brake : simulink/Logic and Bit Operations/Compare To Constant  relop=>  const=0  OutDataTypeStr=boolean  ZeroCross=off
  Compare To Constant : simulink/Logic and Bit Operations/Compare To Constant  relop===  const=3  OutDataTypeStr=boolean  ZeroCross=off
  Compare To Constant1 : simulink/Logic and Bit Operations/Compare To Constant  relop===  const=2  OutDataTypeStr=boolean  ZeroCross=off
  Compare To Constant2 : simulink/Logic and Bit Operations/Compare To Constant  relop===  const=-1  OutDataTypeStr=boolean  ZeroCross=off
  Compare To Constant3 : simulink/Logic and Bit Operations/Compare To Constant  relop===  const=1  OutDataTypeStr=boolean  ZeroCross=off
  Headlights : Constant  Value=0
  High Beams : LampBlock  Icon=HighBeams
  Low Beams : LampBlock  Icon=LowBeams
  Mux1 : Mux  Inputs=6
  Reverse : simulink/Logic and Bit Operations/Compare To Constant  relop=<  const=0  OutDataTypeStr=boolean  ZeroCross=off
  Rotary Switch : RotarySwitchBlock  LabelPosition=Bottom
  Rotary Switch1 : RotarySwitchBlock  LabelPosition=Bottom
  Selector : Selector  InputPortWidth=3  IndexOptions=Index vector (dialog)  Indices=[2]  OutputSizes=1
  Selector1 : Selector  InputPortWidth=3  IndexOptions=Index vector (dialog)  Indices=[3]  OutputSizes=1
  Signal Lights : Constant  Value=0
  Turn Signal Left : LampBlock  Icon=TurnSignalLeft
  Turn Signal Right : LampBlock  Icon=TurnSignalRight
  Light Controls : Outport
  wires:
  Selector1/1 -> Reverse/1
  Reverse/1 -> Mux1/4
  Compare To Constant2/1 -> Mux1/5  "Left"
  Compare To Constant/1 -> Mux1/1  "Highbeam"
  Compare To Constant1/1 -> Mux1/2  "Lowbeam"
  Compare To Constant3/1 -> Mux1/6  "Right"
  Brake/1 -> Mux1/3
  DriverCmd/1 -> Selector1/1, Selector/1
  Selector/1 -> Brake/1
  Mux1/1 -> Light Controls/1
  Headlights/1 -> Compare To Constant1/1, Compare To Constant/1
  Signal Lights/1 -> Compare To Constant3/1, Compare To Constant2/1

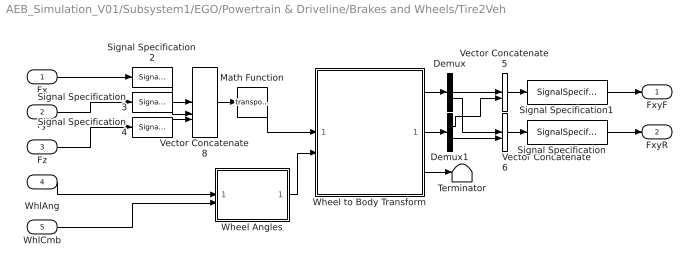
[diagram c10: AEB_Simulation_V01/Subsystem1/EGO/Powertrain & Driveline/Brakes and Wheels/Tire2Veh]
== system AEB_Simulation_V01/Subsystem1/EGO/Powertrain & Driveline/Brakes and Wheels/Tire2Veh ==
  Fx : Inport
  Fy : Inport  Port=2
  Fz : Inport  Port=3
  WhlAng : Inport  Port=4
  WhlCmb : Inport  Port=5
  Demux : Demux  Outputs=[2,2]
  Demux1 : Demux  Outputs=[2,2]
  Math Function : Math  Operator=transpose  SignedPower=on
  Signal Specification : SignalSpecification  Unit=N
  Signal Specification1 : SignalSpecification  Unit=N
  Signal Specification2 : SignalSpecification  Dimensions=4
  Signal Specification3 : SignalSpecification  Dimensions=4
  Signal Specification4 : SignalSpecification  Dimensions=4
  Terminator : Terminator
  Vector Concatenate5 : Concatenate  Mode=Multidimensional array  ConcatenateDimension=2
  Vector Concatenate6 : Concatenate  Mode=Multidimensional array  ConcatenateDimension=2
  Vector Concatenate8 : Concatenate  NumInputs=3  Mode=Multidimensional array  ConcatenateDimension=2
  Wheel Angles : Subsystem
  Wheel to Body Transform : Subsystem
  FxyF : Outport
  FxyR : Outport  Port=2
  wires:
  Wheel Angles/1(Vehicle) -> Wheel to Body Transform/2(WheelAngles)
  Vector Concatenate5/1 -> Signal Specification1/1
  Demux/1 -> Vector Concatenate5/1
  Vector Concatenate8/1 -> Math Function/1
  Signal Specification1/1 -> FxyF/1
  Wheel to Body Transform/1(Fx) -> Demux/1
  Vector Concatenate6/1 -> Signal Specification/1
  Signal Specification4/1 -> Vector Concatenate8/3
  Demux1/2 -> Vector Concatenate6/2
  Wheel to Body Transform/2(Fy) -> Demux1/1
  Fy/1 -> Signal Specification3/1
  Math Function/1 -> Wheel to Body Transform/1(Forces)
  Wheel to Body Transform/3(Fz) -> Terminator/1
  Demux/2 -> Vector Concatenate6/1
  Signal Specification3/1 -> Vector Concatenate8/2
  Signal Specification2/1 -> Vector Concatenate8/1
  Demux1/1 -> Vector Concatenate5/2
  WhlAng/1 -> Wheel Angles/1(Front)
  Fx/1 -> Signal Specification2/1
  Fz/1 -> Signal Specification4/1
  Signal Specification/1 -> FxyR/1
  WhlCmb/1 -> Wheel Angles/2(Camber)

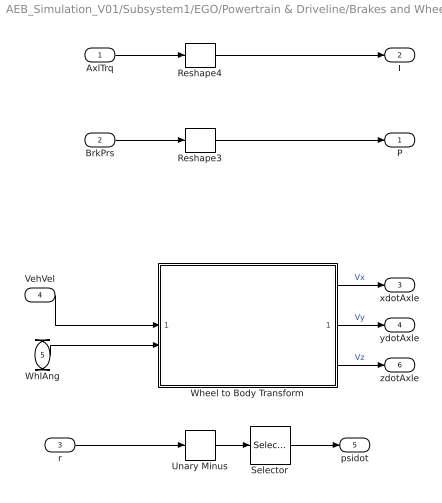
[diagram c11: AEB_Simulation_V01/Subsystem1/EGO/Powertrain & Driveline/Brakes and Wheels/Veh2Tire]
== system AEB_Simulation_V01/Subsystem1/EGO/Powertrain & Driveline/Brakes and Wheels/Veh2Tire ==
  AxlTrq : Inport
  BrkPrs : Inport  Port=2
  r : Inport  Port=3
  VehVel : Inport  Port=4
  WhlAng : Inport  Port=5
  Reshape3 : Reshape
  Reshape4 : Reshape
  Selector : Selector  InputPortWidth=1  IndexOptions=Index vector (dialog)  Indices=[1 1 1 1]  OutputSizes=1
  Unary Minus : UnaryMinus
  Wheel to Body Transform : Subsystem
  P : Outport  VectorParamsAs1DForOutWhenUnconnected=off
  T : Outport  Port=2  VectorParamsAs1DForOutWhenUnconnected=off
  xdotAxle : Outport  Port=3  VectorParamsAs1DForOutWhenUnconnected=off
  ydotAxle : Outport  Port=4  VectorParamsAs1DForOutWhenUnconnected=off
  psidot : Outport  Port=5  VectorParamsAs1DForOutWhenUnconnected=off
  zdotAxle : Outport  Port=6  VectorParamsAs1DForOutWhenUnconnected=off
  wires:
  BrkPrs/1 -> Reshape3/1
  AxlTrq/1 -> Reshape4/1
  Wheel to Body Transform/1(xdotWheel) -> xdotAxle/1  "Vx"
  Wheel to Body Transform/2(ydotWheel) -> ydotAxle/1  "Vy"
  r/1 -> Unary Minus/1
  Reshape4/1 -> T/1
  VehVel/1 -> Wheel to Body Transform/1(VelVeh)
  Wheel to Body Transform/3(zdotWheel) -> zdotAxle/1  "Vz"
  Unary Minus/1 -> Selector/1
  Reshape3/1 -> P/1
  WhlAng/1 -> Wheel to Body Transform/2(WhlAng)
  Selector/1 -> psidot/1

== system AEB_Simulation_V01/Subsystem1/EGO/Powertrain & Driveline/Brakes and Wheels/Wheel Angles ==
  steer : Inport
  camber : Inport  Port=2
  Add1 : Sum
  Add2 : Sum
  Constant1 : Constant  Value=pi
  Constant2 : Constant  Value=[pi;0;pi;0].*0+[0;pi;0;pi].*0
  Constant3 : Constant  Value=ones(1,4).*0
  Reshape : Reshape  OutputDimensionality=Row vector (2-D)
  Reshape1 : Reshape  OutputDimensionality=Row vector (2-D)
  Reshape2 : Reshape  OutputDimensionality=Row vector (2-D)
  Vector Concatenate3 : Concatenate  NumInputs=3  Mode=Multidimensional array
  WhlAngB : Outport  VectorParamsAs1DForOutWhenUnconnected=off
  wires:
  Constant1/1 -> Add2/2
  Add2/1 -> Reshape1/1
  Add1/1 -> Reshape/1
  Reshape2/1 -> Vector Concatenate3/2
  Reshape1/1 -> Vector Concatenate3/1
  Constant3/1 -> Reshape2/1
  camber/1 -> Add2/1
  steer/1 -> Add1/1
  Reshape/1 -> Vector Concatenate3/3
  Vector Concatenate3/1 -> WhlAngB/1
  Constant2/1 -> Add1/2

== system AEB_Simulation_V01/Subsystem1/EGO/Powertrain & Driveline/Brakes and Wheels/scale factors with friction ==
  lamda_mu_x : Inport
  lamda_mu_y : Inport  Port=2
  0 : Constant  Value=[zeros(1,numWheels)]  VectorParams1D=off
  Reshape : Reshape  OutputDimensionality=Row vector (2-D)  OutputDimensions=[1,numWheels]
  Reshape1 : Reshape  OutputDimensionality=Row vector (2-D)  OutputDimensions=[1,numWheels]
  Signal Specification3 : SignalSpecification  Unit=1
  Vector Concatenate : Concatenate  NumInputs=5  Mode=Multidimensional array
  ones : Constant  Value=[ones(23,numWheels)]  VectorParams1D=off
  ones2 : Constant  Value=ones(1,numWheels)  VectorParams1D=off
  lambdas : Outport  Unit=1  VectorParamsAs1DForOutWhenUnconnected=off
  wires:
  lamda_mu_y/1 -> Reshape1/1
  lamda_mu_x/1 -> Reshape/1
  ones2/1 -> Vector Concatenate/1  "lambda_Fz0"
  Vector Concatenate/1 -> Signal Specification3/1
  ones/1 -> Vector Concatenate/5
  0/1 -> Vector Concatenate/4  "lamda_mu_V"
  Reshape1/1 -> Vector Concatenate/3
  Reshape/1 -> Vector Concatenate/2
  Signal Specification3/1 -> lambdas/1

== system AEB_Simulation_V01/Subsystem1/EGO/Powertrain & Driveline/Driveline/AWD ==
  TPowertrain : Inport
  Gear : Inport  Port=2
  AWD : Gain  Gain=[1;1;1;1]./2
  Add : Sum
  Constant : Constant
  Constant1 : Constant  Value=zeros(4,1)
  Multiport Switch : MultiPortSwitch  DataPortOrder=Zero-based contiguous  zeroidx=on
  Unary Minus : UnaryMinus
  TAxles : Outport  VectorParamsAs1DForOutWhenUnconnected=off
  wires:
  TPowertrain/1 -> AWD/1
  Multiport Switch/1 -> TAxles/1
  Add/1 -> Multiport Switch/1
  Constant1/1 -> Multiport Switch/3
  AWD/1 -> Unary Minus/1, Multiport Switch/4
  Constant/1 -> Add/2
  Gear/1 -> Add/1
  Unary Minus/1 -> Multiport Switch/2

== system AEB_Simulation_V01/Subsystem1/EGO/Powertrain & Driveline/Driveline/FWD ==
  TPowertrain : Inport
  Gear : Inport  Port=2
  Add : Sum
  Constant : Constant
  Constant1 : Constant  Value=zeros(4,1)
  FWD : Gain  Gain=[1;1;0;0]
  Multiport Switch : MultiPortSwitch  DataPortOrder=Zero-based contiguous  zeroidx=on
  Unary Minus : UnaryMinus
  TAxles : Outport  VectorParamsAs1DForOutWhenUnconnected=off
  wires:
  TPowertrain/1 -> FWD/1
  Multiport Switch/1 -> TAxles/1
  Add/1 -> Multiport Switch/1
  Constant1/1 -> Multiport Switch/3
  FWD/1 -> Unary Minus/1, Multiport Switch/4
  Constant/1 -> Add/2
  Gear/1 -> Add/1
  Unary Minus/1 -> Multiport Switch/2

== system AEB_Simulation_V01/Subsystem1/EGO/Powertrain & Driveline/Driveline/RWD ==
  TPowertrain : Inport
  Gear : Inport  Port=2
  Add : Sum
  Constant : Constant
  Constant1 : Constant  Value=zeros(4,1)
  Multiport Switch : MultiPortSwitch  DataPortOrder=Zero-based contiguous  zeroidx=on
  RWD : Gain  Gain=[0;0;1;1]
  Unary Minus : UnaryMinus
  TAxles : Outport  VectorParamsAs1DForOutWhenUnconnected=off
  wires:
  RWD/1 -> Unary Minus/1, Multiport Switch/4
  TPowertrain/1 -> RWD/1
  Unary Minus/1 -> Multiport Switch/2
  Multiport Switch/1 -> TAxles/1
  Gear/1 -> Add/1
  Constant/1 -> Add/2
  Add/1 -> Multiport Switch/1
  Constant1/1 -> Multiport Switch/3

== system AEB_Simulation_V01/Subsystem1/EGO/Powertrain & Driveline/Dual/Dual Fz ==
  In1 : Inport
  Add : Sum
  Bus Selector : BusSelector  OutputSignals=VehFdbk
  Bus Selector6 : BusSelector  OutputSignals=BdyFrm.Forces.Tires.FrntTires.Lft.Fz,BdyFrm.Forces.Tires.FrntTires.Rght.Fz,BdyFrm.Forces.Tires.RearTires.Lft.Fz,BdyFrm.Forces.Tires.RearTires.Rght.Fz
  Cont LPF : autolibutils/Cont LPF  wc=100*2*pi  AbsoluteTolerance=auto  aMode=2
  Saturation : Saturate  UpperLimit=10e3  LowerLimit=100  ZeroCross=off
  Unsprung Mass : Constant  Value=[0 0 80 80].*9.81
  Vector Concatenate : Concatenate  NumInputs=4
  Out1 : Outport  VectorParamsAs1DForOutWhenUnconnected=off
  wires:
  In1/1 -> Bus Selector/1
  Saturation/1 -> Cont LPF/1
  Cont LPF/1 -> Add/1
  Vector Concatenate/1 -> Saturation/1
  Bus Selector6/2 -> Vector Concatenate/2  "<Fz>"
  Bus Selector6/1 -> Vector Concatenate/1  "<Fz>"
  Bus Selector6/3 -> Vector Concatenate/3  "<Fz>"
  Bus Selector6/4 -> Vector Concatenate/4  "<Fz>"
  Add/1 -> Out1/1
  Unsprung Mass/1 -> Add/2
  Bus Selector/1 -> Bus Selector6/1  "<VehFdbk>"

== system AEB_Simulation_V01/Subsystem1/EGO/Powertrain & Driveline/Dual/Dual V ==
  In1 : Inport
  Bus Selector : BusSelector  OutputSignals=VehFdbk
  Bus Selector1 : BusSelector  OutputSignals=BdyFrm.FrntAxl.Lft.Vel.xdot,BdyFrm.FrntAxl.Lft.Vel.ydot,BdyFrm.FrntAxl.Lft.Vel.zdot  OutputAsBus=on
  Bus Selector2 : BusSelector  OutputSignals=BdyFrm.FrntAxl.Rght.Vel.xdot,BdyFrm.FrntAxl.Rght.Vel.ydot,BdyFrm.FrntAxl.Rght.Vel.zdot  OutputAsBus=on
  Bus Selector4 : BusSelector  OutputSignals=BdyFrm.RearAxl.Lft.Vel.xdot,BdyFrm.RearAxl.Lft.Vel.ydot,BdyFrm.RearAxl.Lft.Vel.zdot  OutputAsBus=on
  Bus Selector5 : BusSelector  OutputSignals=BdyFrm.RearAxl.Rght.Vel.xdot,BdyFrm.RearAxl.Rght.Vel.ydot,BdyFrm.RearAxl.Rght.Vel.zdot  OutputAsBus=on
  Bus to Vector{5..8} (4 alike) : BusToVector
  Vector Concatenate2 : Concatenate  NumInputs=4  Mode=Multidimensional array  ConcatenateDimension=2
  Out1 : Outport  VectorParamsAs1DForOutWhenUnconnected=off
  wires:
  Bus to Vector6/1 -> Vector Concatenate2/2
  Bus Selector2/1 -> Bus to Vector6/1
  Bus to Vector8/1 -> Vector Concatenate2/4
  Bus Selector4/1 -> Bus to Vector7/1
  Bus to Vector5/1 -> Vector Concatenate2/1
  Bus Selector1/1 -> Bus to Vector5/1
  Bus Selector/1 -> Bus Selector1/1, Bus Selector2/1, Bus Selector4/1, Bus Selector5/1  "<VehFdbk>"
  Bus Selector5/1 -> Bus to Vector8/1
  Bus to Vector7/1 -> Vector Concatenate2/3
  Vector Concatenate2/1 -> Out1/1
  In1/1 -> Bus Selector/1

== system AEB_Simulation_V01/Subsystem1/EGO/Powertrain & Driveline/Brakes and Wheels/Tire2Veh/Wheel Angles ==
  Front : Inport
  Camber : Inport  Port=2
  Add1 : Sum
  Add2 : Sum
  Constant1 : Constant  Value=pi
  Constant2 : Constant  Value=[pi;0;pi;0].*0+[0;pi;0;pi].*.0
  Constant3 : Constant  Value=ones(1,4).*0
  Reshape : Reshape  OutputDimensionality=Row vector (2-D)
  Reshape1 : Reshape  OutputDimensionality=Row vector (2-D)
  Reshape2 : Reshape  OutputDimensionality=Row vector (2-D)
  Vector Concatenate3 : Concatenate  NumInputs=3  Mode=Multidimensional array
  Vehicle : Outport  VectorParamsAs1DForOutWhenUnconnected=off
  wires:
  Constant1/1 -> Add2/2
  Reshape/1 -> Vector Concatenate3/3
  Reshape2/1 -> Vector Concatenate3/2
  Front/1 -> Add1/1
  Add2/1 -> Reshape1/1
  Add1/1 -> Reshape/1
  Constant3/1 -> Reshape2/1
  Reshape1/1 -> Vector Concatenate3/1
  Constant2/1 -> Add1/2
  Camber/1 -> Add2/1
  Vector Concatenate3/1 -> Vehicle/1

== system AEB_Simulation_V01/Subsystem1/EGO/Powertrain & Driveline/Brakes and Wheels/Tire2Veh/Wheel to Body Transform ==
  Forces : Inport  PortDimensions=[3,1]  Partition=on  PartitionDimension=2  PartitionWidth=1  PartitionOffset=0
  WheelAngles : Inport  Port=2  Partition=on  PartitionDimension=2  PartitionWidth=1  PartitionOffset=0
  Demux1 : Demux  Outputs=3
  Divide1 : Product  Inputs=**  Multiplication=Matrix(*)
  For Each : ForEach  DisableCoverage=on
  Rotation Angles to Direction Cosine Matrix : sharedtransform/Rotation Angles to Direction Cosine Matrix  rotationOrder=ZYX  aMode=2
  Selector : Selector  InputPortWidth=3  IndexOptions=Index vector (dialog)  Indices=[3 2 1]  OutputSizes=1
  Fx : Outport  ConcatenationDimension=1  VectorParamsAs1DForOutWhenUnconnected=off
  Fy : Outport  Port=2  ConcatenationDimension=1  VectorParamsAs1DForOutWhenUnconnected=off
  Fz : Outport  Port=3  ConcatenationDimension=1  VectorParamsAs1DForOutWhenUnconnected=off
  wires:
  Divide1/1 -> Demux1/1
  Demux1/1 -> Fx/1
  Demux1/2 -> Fy/1
  Demux1/3 -> Fz/1
  Rotation Angles to Direction Cosine Matrix/1 -> Divide1/1
  Forces/1 -> Divide1/2
  WheelAngles/1 -> Selector/1
  Selector/1 -> Rotation Angles to Direction Cosine Matrix/1

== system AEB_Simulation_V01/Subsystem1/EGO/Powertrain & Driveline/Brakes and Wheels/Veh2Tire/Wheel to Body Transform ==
  VelVeh : Inport  Partition=on  PartitionDimension=2  PartitionWidth=1  PartitionOffset=0
  WhlAng : Inport  Port=2  Partition=on  PartitionDimension=2  PartitionWidth=1  PartitionOffset=0
  Demux1 : Demux  Outputs=3
  Divide1 : Product  Inputs=**  Multiplication=Matrix(*)
  For Each : ForEach  DisableCoverage=on
  Rotation Angles to Direction Cosine Matrix : sharedtransform/Rotation Angles to Direction Cosine Matrix  rotationOrder=ZYX  aMode=2
  Selector : Selector  InputPortWidth=3  IndexOptions=Index vector (dialog)  Indices=[3 2 1]  OutputSizes=1
  xdotWheel : Outport  ConcatenationDimension=1  VectorParamsAs1DForOutWhenUnconnected=off
  ydotWheel : Outport  Port=2  ConcatenationDimension=1  VectorParamsAs1DForOutWhenUnconnected=off
  zdotWheel : Outport  Port=3  ConcatenationDimension=1  VectorParamsAs1DForOutWhenUnconnected=off
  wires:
  Divide1/1 -> Demux1/1
  Demux1/1 -> xdotWheel/1
  Demux1/2 -> ydotWheel/1
  Demux1/3 -> zdotWheel/1
  Rotation Angles to Direction Cosine Matrix/1 -> Divide1/1
  VelVeh/1 -> Divide1/2
  WhlAng/1 -> Selector/1
  Selector/1 -> Rotation Angles to Direction Cosine Matrix/1

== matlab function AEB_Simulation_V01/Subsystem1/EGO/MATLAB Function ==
function [acc, dec]  = fcn(AEB)

acc = 1.0;
dec = 0.0;

if (AEB == 1.0)
    acc = 1.0;
    dec = 0.0;
end

if (AEB == 2.0)
    acc = 0.5;
    dec = 0.0;
end

if (AEB == 3.0)
    acc = 0.1;
    dec = 0.0;
end

if (AEB == 4.0)
    acc = 0.0;
    dec = 1.0;
end
